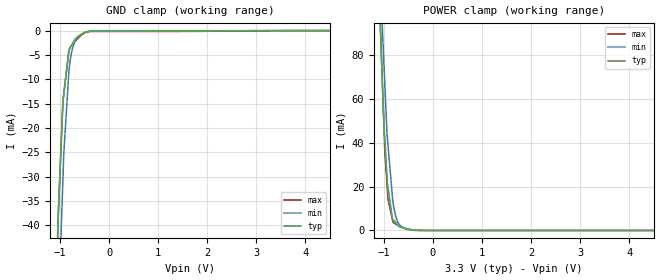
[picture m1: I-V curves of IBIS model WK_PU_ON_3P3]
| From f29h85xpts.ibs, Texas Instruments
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|RECEIVER_MODE_3P3; RECEIVER_MODE
|   Model Cell WK_PU_ON_3P3
|WK_PU_ON_3P3
[Model]   WK_PU_ON_3P3
Model_type   Input
Polarity   Non-Inverting
Vinl = 0.8
Vinh = 2
|   typ   min   max
C_comp   0.36pF   0.33pF   0.38pF
[Model Spec]
Vinl   0.8   0.8   0.8
Vinh   2   2   2
[Temperature Range]   25   155   -40
[Voltage Range]   3.3   2.8   3.63
| Nom Voltages:
|   VDD=1.23, VDDS=3.3, VSS=0
| Min Voltages:
|   VDD=1.08, VDDS=2.8, VSS=0
| Max Voltages:
|   VDD=1.32, VDDS=3.63, VSS=0
[Power Clamp Reference]   3.3   2.8   3.63
[GND Clamp Reference]   0   0   0
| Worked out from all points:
|   GND clamp passes 1 mA (typ) near -0.60 V on its own axis
|   POWER clamp passes 1 mA (typ) near -0.57 V on its own axis
[GND Clamp]
|   Voltage   I(typ)   I(min)   I(max)
-3.3V     -1.461A    -1.198A    -2.144A
-1.047V   -41.9mA    -64.15mA   -40.67mA
-1.024V   -34.01mA   -55.26mA   -34.97mA
-945.8mV  -15.24mA   -31.6mA    -15.56mA
-940.1mV  -14.71mA   -29.85mA   -14.13mA
-925.2mV  -13.34mA   -25.33mA   -12.91mA
-824.4mV  -4.071mA   -9.058mA   -4.694mA
-813.8mV  -3.883mA   -7.757mA   -3.825mA
-758mV    -2.896mA   -4.105mA   -2.924mA
-702.3mV  -1.913mA   -2.324mA   -2.251mA
-493.3mV  -316.9uA   -387.8uA   -465.8uA
6.6V      0A         0A         0A
[POWER Clamp]
|   Voltage   I(typ)   I(min)   I(max)
-3.3V     1.933A     2.239A     2.093A
-1.07V    91.62mA    120.9mA    92.59mA
-1.035V   70.42mA    95.89mA    70.71mA
-1.024V   63.33mA    88.74mA    63.38mA
-978.6mV  41.47mA    65.94mA    35.65mA
-934.4mV  24.28mA    43.68mA    20.54mA
-915.2mV  19.67mA    38.7mA     13.98mA
-819.6mV  5.174mA    13.9mA     4.379mA
-758mV    3.597mA    6.477mA    2.859mA
-687.7mV  1.799mA    2.771mA    2.056mA
-274.8mV  29.35uA    31.91uA    56.46uA
6.6V      0A         0A         0A
